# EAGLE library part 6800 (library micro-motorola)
MICROCONTROLLER/MEMORY DEVICE
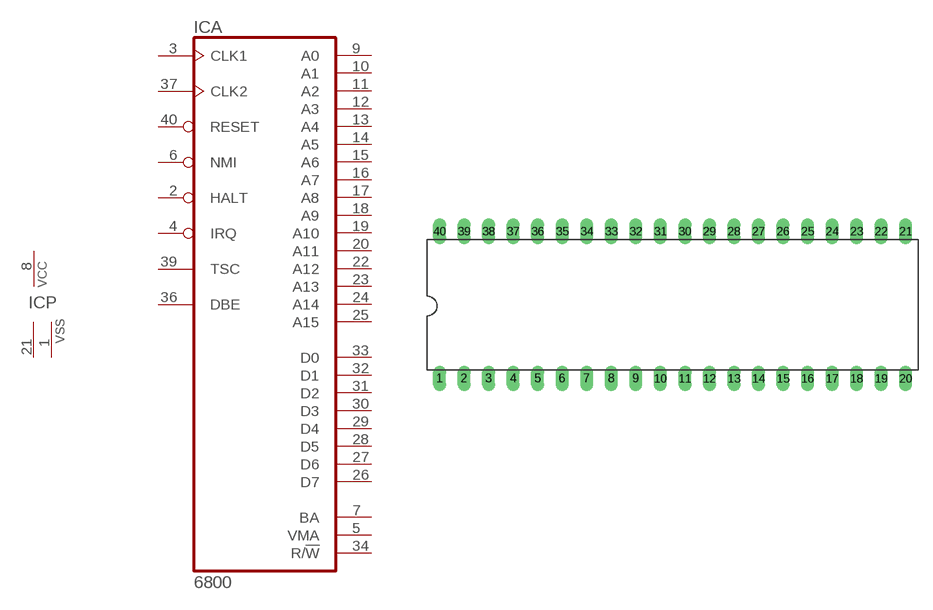
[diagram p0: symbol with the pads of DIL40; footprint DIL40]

Designator prefix IC; gates A=6800 P=PWR2VSS

## 6800 (MF: NTE ELECTRONICS; MPN: NTE6800; OC_FARNELL: unknown; OC_NEWARK: 31C5317)  [DIL40]
1  P:VSS  pwr
2  A:HALT  in
3  A:CLK1  in
4  A:IRQ  in
5  A:VMA  out
6  A:NMI  in
7  A:BA  out
8  P:VCC  pwr
9  A:A0  out
10  A:A1  out
11  A:A2  out
12  A:A3  out
13  A:A4  out
14  A:A5  out
15  A:A6  out
16  A:A7  out
17  A:A8  out
18  A:A9  out
19  A:A10  out
20  A:A11  out
21  P:VSS  pwr
22  A:A12  out
23  A:A13  out
24  A:A14  out
25  A:A15  out
26  A:D7
27  A:D6
28  A:D5
29  A:D4
30  A:D3
31  A:D2
32  A:D1
33  A:D0
34  A:R/!W  out
36  A:DBE  in
37  A:CLK2  in
39  A:TSC  in
40  A:RESET  in

## Footprint DIL40 (pad centres in mm)
Dual In Line Package
drill 0.813 long: 1 -24.13,-7.62; 2 -21.59,-7.62; 3 -19.05,-7.62; 4 -16.51,-7.62; 5 -13.97,-7.62; 6 -11.43,-7.62; 7 -8.89,-7.62; 8 -6.35,-7.62; 9 -3.81,-7.62; 10 -1.27,-7.62; 11 1.27,-7.62; 12 3.81,-7.62; 13 6.35,-7.62; 14 8.89,-7.62; 15 11.43,-7.62; 16 13.97,-7.62; 17 16.51,-7.62; 18 19.05,-7.62; 19 21.59,-7.62; 20 24.13,-7.62; 21 24.13,7.62; 22 21.59,7.62; 23 19.05,7.62; 24 16.51,7.62; 25 13.97,7.62; 26 11.43,7.62; 27 8.89,7.62; 28 6.35,7.62; 29 3.81,7.62; 30 1.27,7.62; 31 -1.27,7.62; 32 -3.81,7.62; 33 -6.35,7.62; 34 -8.89,7.62; 35 -11.43,7.62; 36 -13.97,7.62; 37 -16.51,7.62; 38 -19.05,7.62; 39 -21.59,7.62; 40 -24.13,7.62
